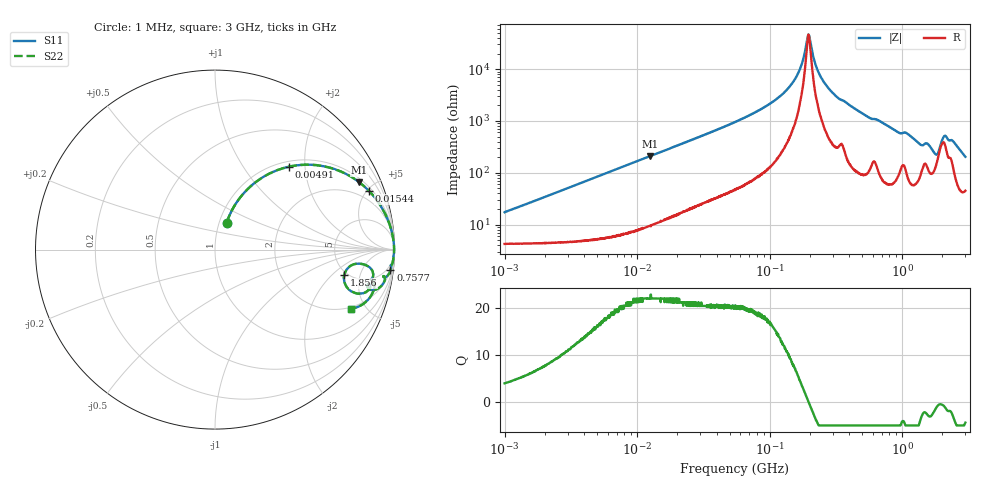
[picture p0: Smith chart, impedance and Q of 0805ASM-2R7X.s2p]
!s-Parameter Generated by FASTRON Sdn. Bhd.
!FASTRON P/N : 0805AS-2R7X
!Keysight Technologies: E4991B_MY54100416_A.01.15
!Date: Fri Jun 19 14:54:27 2026
!Version  :Rev00  Fri Jun 19 14:54:27 2026
!Data & Calibration Information:
!Freq  S11  S21  S12  S22
!PortZ  Port1:50+j0  Port2:50+j0
!When reading reference impedance value at option line is always used.
! Remarks : This data is being provided solely for informational purposes.
# Hz S dB R 50
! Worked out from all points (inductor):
!   1601 points, 1 MHz to 3 GHz, reference 50 ohm
!   read as one part in series: L = 2.69 uH near 1.041 MHz
!   highest Q = 22 at 12.52 MHz (marker M1), where L = 2.67 uH
!   self-resonance near 196.2 MHz
!   S11 on the Smith chart (normalised r, x): 1 MHz: 1.08, +0.34; 4.91 MHz: 1.10, +1.65; 15.44 MHz: 1.23, +5.16; 757.7 MHz: 2, -17; 1.856 GHz: 4.69, -2.87; 3 GHz: 1.90, -3.96
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1000000  -15.70 66.7  -0.47 -9.2  -0.47 -9.2  -15.70 66.7
3804036  -5.63 54.3  -1.79 -31.4  -1.79 -31.4  -5.63 54.3
4909959  -4.17 48.3  -2.53 -38.1  -2.53 -38.1  -4.17 48.3
1.251602e7  -1.04 25.0  -7.48 -62.4  -7.48 -62.4  -1.04 25.0
1.447069e7  -0.82 22.0  -8.51 -65.4  -8.51 -65.4  -0.82 22.0
1.544333e7  -0.73 20.8  -8.99 -66.6  -8.99 -66.6  -0.73 20.8
5.504702e7  -0.09 5.9  -19.70 -81.3  -19.70 -81.3  -0.09 5.9
1.250659e8  -0.03 1.7  -30.40 -83.6  -30.40 -83.6  -0.03 1.7
1.63867e8  -0.02 0.7  -38.40 -79.1  -38.40 -79.1  -0.02 0.7
1.766402e8  -0.02 0.4  -42.80 -72.7  -42.80 -72.7  -0.02 0.4
1.942587e8  -0.02 0.0  -52.80 -21.1  -52.80 -21.1  -0.02 0.0
2.001795e8  -0.02 -0.1  -52.10 28.3  -52.10 28.3  -0.02 -0.1
2.083556e8  -0.02 -0.2  -47.30 59.5  -47.30 59.5  -0.02 -0.2
2.373059e8  -0.02 -0.7  -38.10 78.9  -38.10 78.9  -0.02 -0.7
2.987278e8  -0.03 -1.6  -30.90 82.6  -30.90 82.6  -0.03 -1.6
7.576891e8  -0.14 -6.7  -18.60 79.0  -18.60 79.0  -0.14 -6.7
7.925923e8  -0.15 -7.2  -18.00 78.5  -18.00 78.5  -0.15 -7.2
1.687342e9  -1.40 -16.7  -10.30 52.9  -10.30 52.9  -1.40 -16.7
1.855641e9  -2.69 -11.1  -10.10 26.8  -10.10 26.8  -2.69 -11.1
2.113475e9  -1.08 -7.5  -15.40 42.8  -15.40 42.8  -1.08 -7.5
2.543347e9  -0.80 -14.8  -11.60 63.1  -11.60 63.1  -0.80 -14.8
3e9  -1.65 -23.4  -7.81 53.8  -7.81 53.8  -1.65 -23.4
